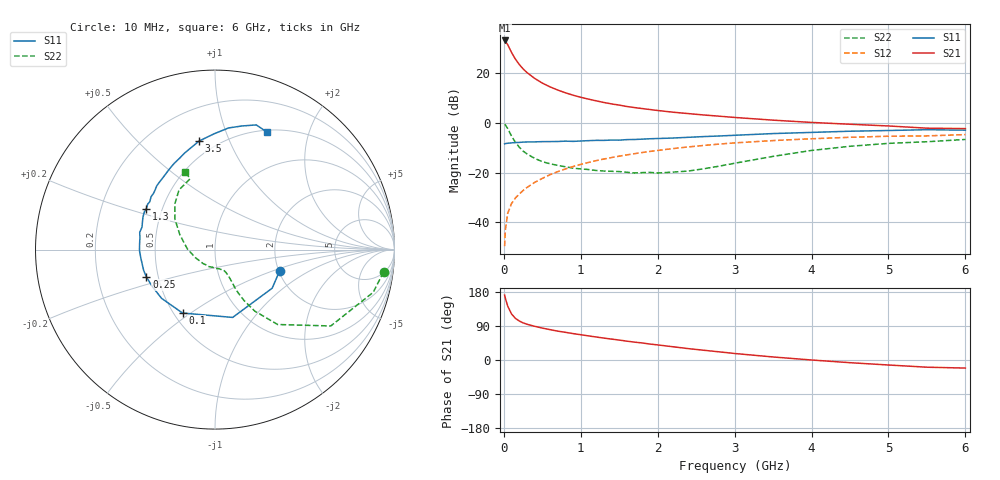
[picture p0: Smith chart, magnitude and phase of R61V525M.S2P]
! SIEMENS Small Signal Semiconductors
! BFR193
! Si NPN RF Bipolar Junction Transistor in SOT23
! VCE = 1.5 V  IC = 25 mA
! Common Emitter S-Parameters:  May  1996
# GHz  S  MA  R  50
!  f  S11  S21  S12  S22
! GHz  MAG  ANG  MAG  ANG  MAG  ANG  MAG  ANG
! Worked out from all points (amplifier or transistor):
!   36 points, 10 MHz to 6 GHz, reference 50 ohm
!   highest |S21| = 33.2 dB at 10 MHz (marker M1)
!   |S21| within 3 dB of that: start of sweep to 70.74 MHz
!   unconditionally stable (mu >= 1): 468.1 MHz to 2.021 GHz
!   at 250 MHz: K = 0.88, MSG = 24.5 dB, |S12| = -27.2 dB
!   at 1.4 GHz: K = 1.02, MAG = 9.8 dB, |S12| = -13.9 dB
!   at 6 GHz: K = 0.96, MSG = 1.2 dB, |S12| = -4.7 dB
!   S11 on the Smith chart (normalised r, x): 10 MHz: 2.03, -0.55; 100 MHz: 0.55, -0.47; 250 MHz: 0.43, -0.16; 1.3 GHz: 0.41, +0.23; 3.5 GHz: 0.40, +0.78; 6 GHz: 0.52, +1.40
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0.01  0.3793 -18.0  45.88 171.3  0.0033 80.6  0.9472 -7.6
0.02  0.3844 -34.0  44.48 162.8  0.007 80.8  0.9132 -15.1
0.05  0.3905 -75.4  37.71 142.3  0.0151 70.9  0.7728 -33.4
0.1  0.397 -117.1  26.32 121.5  0.0238 63.9  0.5441 -50.1
0.15  0.4029 -137.6  19.31 109.9  0.0308 62.9  0.4082 -57.1
0.2  0.4055 -149.8  15.12 103.0  0.0368 65.0  0.3263 -60.3
0.25  0.4117 -158.3  12.28 98.0  0.0436 66.2  0.2722 -61.9
0.3  0.4141 -163.9  10.37 94.4  0.0501 68.0  0.2382 -62.4
0.4  0.4158 -173.4  7.913 89.0  0.0634 69.3  0.1941 -62.5
0.5  0.4209 -179.3  6.354 84.2  0.0765 70.4  0.166 -62.9
0.6  0.4214 175.2  5.335 80.1  0.0908 69.8  0.1508 -63.7
0.7  0.4233 171.1  4.608 76.2  0.1046 69.3  0.1399 -64.6
0.9  0.4256 162.9  3.624 69.7  0.1328 67.8  0.1229 -67.4
1.1  0.4401 155.8  3.02 63.6  0.1603 66.0  0.1154 -73.5
1.3  0.4456 149.1  2.586 57.8  0.1878 63.3  0.1076 -80.3
1.7  0.4645 137.4  2.04 47.1  0.2407 58.0  0.0984 -99.0
2.2  0.4972 125.0  1.646 34.9  0.305 50.5  0.1024 -130.7
2.8  0.5467 111.0  1.369 21.5  0.3756 41.2  0.1348 -172.3
3.5  0.6115 98.3  1.139 8.0  0.4418 29.9  0.2124 157.1
4.5  0.6818 83.7  0.942 -7.1  0.5148 15.7  0.3392 131.2
5.5  0.7317 71.7  0.785 -19.0  0.5489 1.7  0.4184 109.4
6  0.7163 66.3  0.77 -21.3  0.5831 -2.4  0.4654 110.8
